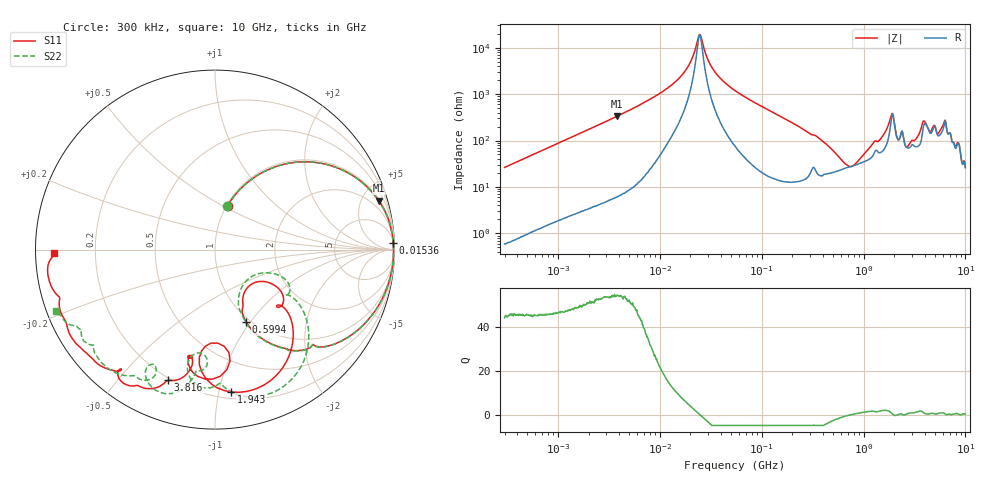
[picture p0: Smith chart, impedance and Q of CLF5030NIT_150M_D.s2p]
! S-Parameter Data Generated by TDK Corporation
! Copyright(C) 2019 TDK Corporation.
! All Rights Reserved.
! TDK P/N: CLF5030NIT-150M-D (Inductor)
! Property: L=15uH at 100kHz
! Size(LxWxT): 5.3x5x2.7mm
! Model Type: s2p (Touchstone File Format Version 1.0)
! Frequency: DC=Yes Start=0.3MHz Stop=10000MHz 802points Log-sweep
! Model Generated on May 10, 2019
! Port Assignments:
!  1 ---@@@--- 2
! Applicable Conditions:
!  Temperature = 25 degC
!  DC Bias Current = 0 A
!  Small Signal Operation
! Terms and conditions regarding TDK Simulation Models
! (1)This simulation model is being provided solely for informational purposes. Please refer to the specifications of the products in terms of detailed characteristics of such products.
! (2)In no event shall TDK Corporation of any of its subsidiaries be liable for any loss or damage arising, directly or indirectly,
!  From any information contained in this simulation model, including, but not limited to loss or damages arising from any inaccuracies, omissions or errors in connection with such information.
! (3)Any and all copyrights on this simulation model are owned by TDK Corporation.
!  Duplication or redistribution of this simulation model without prior written permission from TDK Corporation is prohibited.
! (4)This simulation model is subject to any modification or change without any prior notice.
! (5)Neither TDK Corporation nor any of its subsidiaries shall make any warranty, express or implied,
!  Including but not limited to the correctness, implied warranties of merchantability and fitness for a particular purpose with respect to this simulation models.
! (6)The use of this simulation model shall be deemed to have consented to the terms and conditions hereof.
# Hz S MA R 50
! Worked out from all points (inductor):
!   801 points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, 300 kHz to 10 GHz, reference 50 ohm
!   read as one part in series: L = 14 uH near 318.3 kHz
!   highest Q = 54.4 at 3.777 MHz (marker M1), where L = 13.9 uH
!   self-resonance near 24.42 MHz
!   S11 on the Smith chart (normalised r, x): 300 kHz: 1.01, +0.53; 15.36 MHz: 10, +56; 599.4 MHz: 0.95, -0.95; 1.943 GHz: 0.25, -1.09; 3.816 GHz: 0.19, -0.69; 10 GHz: 0.05, -0.01
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300000  0.2541 74.1  0.9615 -14.7  0.9612 -14.7  0.254 74.1
1713600  0.8207 33.6  0.5549 -55.2  0.5548 -55.2  0.8208 33.6
3777497  0.9521 16.6  0.2886 -72.3  0.2886 -72.3  0.9521 16.6
9671944  0.9906 5.4  0.1005 -82.2  0.1005 -82.2  0.9906 5.4
1.535588e7  0.9939 2.0  0.04612 -81.7  0.04614 -81.7  0.9939 2.0
1.968205e7  0.9945 0.4  0.0219 -75.9  0.02194 -75.9  0.9946 0.4
2.473055e7  0.9947 -1.0  0.005186 0.7  0.00519 0.7  0.9948 -1.0
3.337006e7  0.9943 -3.0  0.02908 76.8  0.02907 76.9  0.9944 -3.0
5.477226e7  0.9912 -7.0  0.08315 79.4  0.08317 79.4  0.9913 -7.0
1.563148e8  0.9461 -23.0  0.2874 64.6  0.2873 64.6  0.9462 -23.1
3.126428e8  0.765 -44.0  0.5273 36.2  0.5272 36.2  0.766 -44.2
5.99416e8  0.4395 -66.7  0.7328 -0.5  0.7329 -0.5  0.4381 -67.1
8.872678e8  0.2779 -48.6  0.7387 -30.8  0.7388 -30.8  0.2478 -48.4
1.149233e9  0.3736 -31.1  0.6627 -55.6  0.6628 -55.6  0.3361 -22.9
1.767019e9  0.7719 -62.5  0.2783 -106.0  0.2785 -106.0  0.7784 -49.5
1.942751e9  0.7983 -83.5  0.1425 -69.5  0.1426 -69.6  0.8589 -68.0
2.720446e9  0.6111 -103.4  0.3843 -84.0  0.3824 -84.1  0.5841 -99.7
3.34571e9  0.6674 -101.4  0.2827 -125.2  0.2817 -125.2  0.7065 -99.3
3.816223e9  0.7732 -109.7  0.1176 -139.0  0.1169 -138.6  0.8356 -106.5
5.445625e9  0.8493 -127.9  0.1295 -135.6  0.13 -135.5  0.8429 -123.5
6.253087e9  0.9121 -135.6  0.04843 -146.4  0.04801 -146.6  0.89 -136.6
1e10  0.8991 -178.6  0.03562 -89.8  0.03545 -89.9  0.9497 -158.9
